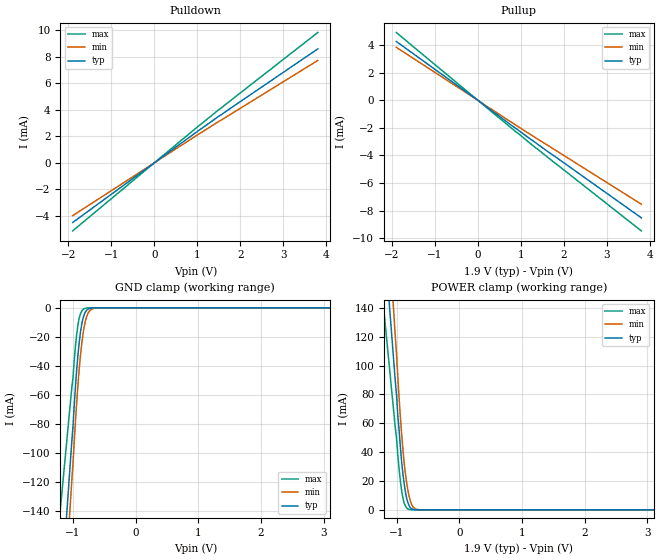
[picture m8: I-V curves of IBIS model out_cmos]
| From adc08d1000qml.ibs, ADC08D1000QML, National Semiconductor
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[Model]   out_cmos
Model_type Output
Vref=0.000E+00
Rref=1.000E+06
Cref=0.000E+00
Vmeas=9.500E-01
C_comp   4.580E-13   4.580E-13   4.580E-13
[Voltage Range]   1.900E+00   1.800E+00   2.000E+00
[POWER Clamp Reference]   1.900E+00   1.800E+00   2.000E+00
[GND Clamp Reference]   0.000E+00   0.000E+00   0.000E+00
[Pullup Reference]   1.900E+00   1.800E+00   2.000E+00
[Pulldown Reference]   0.000E+00   0.000E+00   0.000E+00
[Temperature Range]   25   125   -55
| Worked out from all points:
|   slope of the pulldown table from 0 to 0.285 V, typ, clamps not added: 421 ohm
|   slope of the pullup table from 0 to 0.285 V, typ, clamps not added: 425 ohm
|   GND clamp passes 1 mA (typ) near -0.76 V on its own axis
|   POWER clamp passes 1 mA (typ) near -0.77 V on its own axis
[GND Clamp]
-1.9V     -637mA     -718.2mA   -458.2mA
-1.02V    -92.45mA   -119.6mA   -55.37mA
-1V       -81.45mA   -106.9mA   -48.13mA
-960mV    -53.9mA    -77.82mA   -25.95mA
-920mV    -32.03mA   -52.55mA   -11.45mA
-880mV    -16.47mA   -32.56mA   -3.999mA
-860mV    -11.22mA   -24.46mA   -2.187mA
-820mV    -4.556mA   -12.7mA    -577.6uA
-780mV    -1.604mA   -5.816mA   -153.6uA
-740mV    -508.8uA   -2.349mA   -49.52uA
-620mV    -37.21uA   -143uA     -15.23uA
3.8V      0A         0A         0A
[Power Clamp]
-1.9V     582.5mA    720.3mA    450.5mA
-1.02V    89.29mA    120.2mA    56.91mA
-1V       79.39mA    107.8mA    49.45mA
-980mV    65.3mA     92.37mA    38.32mA
-960mV    55.6mA     78.06mA    28.52mA
-920mV    33.96mA    53.32mA    13.68mA
-880mV    18.6mA     33.31mA    4.797mA
-820mV    5.087mA    13.65mA    591uA
-780mV    1.494mA    6.171mA    111.7uA
-740mV    394.1uA    2.237mA    25.33uA
-640mV    47.88uA    103.3uA    7.025uA
3.8V      0A         0A         0A
[Pullup]
-1.9V     4.276mA    3.852mA    4.926mA
23.84nV   0A         0A         0A
1.34V     -3.077mA   -2.716mA   -3.44mA
3.8V      -8.531mA   -7.541mA   -9.477mA
[Pulldown]
-1.9V     -4.509mA   -3.992mA   -5.141mA
1.08V     2.56mA     2.274mA    2.923mA
1.52V     3.568mA    3.172mA    4.069mA
3.8V      8.605mA    7.734mA    9.847mA
[Ramp]
dV/dt_f   1.1504E-01/3.0910E-10   9.7636E-02/3.0870E-10   1.3422E-01/3.103E-10
dV/dt_r   1.1504E-01/3.2332E-10   9.7636E-02/3.2500E-10   1.3422E-01/3.1906E-10
R_load = 50
